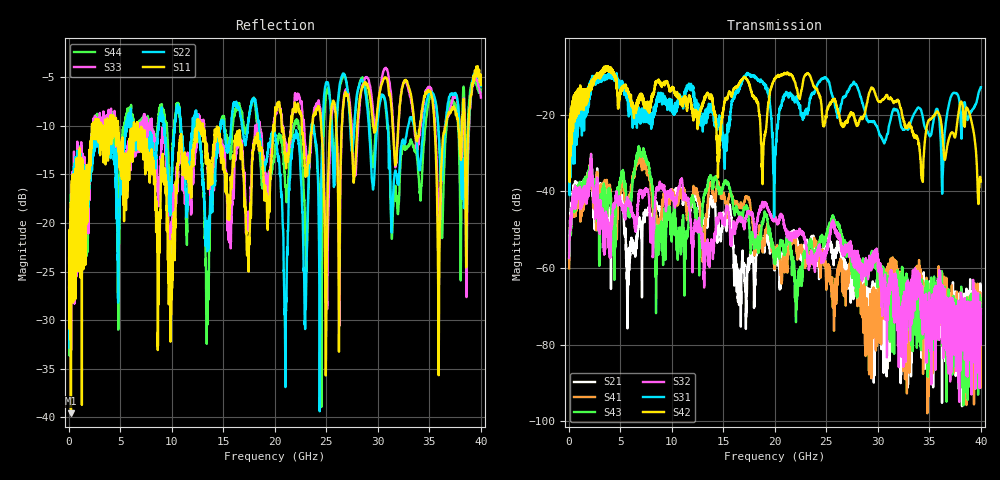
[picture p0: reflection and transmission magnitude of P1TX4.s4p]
!Agilent Technologies,N5245A,MY49151084,A.09.20.08
!Agilent N5245A: A.09.20.08
!Date: Thursday, March 01, 2012 14:23:38
!Correction: S11(Full 4 Port(1,2,3,4))
!S12(Full 4 Port(1,2,3,4))
!S13(Full 4 Port(1,2,3,4))
!S14(Full 4 Port(1,2,3,4))
!S21(Full 4 Port(1,2,3,4))
!S22(Full 4 Port(1,2,3,4))
!S23(Full 4 Port(1,2,3,4))
!S24(Full 4 Port(1,2,3,4))
!S31(Full 4 Port(1,2,3,4))
!S32(Full 4 Port(1,2,3,4))
!S33(Full 4 Port(1,2,3,4))
!S34(Full 4 Port(1,2,3,4))
!S41(Full 4 Port(1,2,3,4))
!S42(Full 4 Port(1,2,3,4))
!S43(Full 4 Port(1,2,3,4))
!S44(Full 4 Port(1,2,3,4))
!S4P File: Measurements: <S11,S12,S13,S14>,
!<S21,S22,S23,S24>,
!<S31,S32,S33,S34>,
!<S41,S42,S43,S44>:
# Hz S  dB  R 50
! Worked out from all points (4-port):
!   3996 points, 50 MHz to 40 GHz, reference 50 ohm
!   strongest paths, dB at 50 MHz, 10.04 GHz, 20.03 GHz, 30.02 GHz, 40 GHz:
!     S42: -25.4, -13.1, -10.5, -16.3, -37.4
!     S31: -26.4, -18.4, -30.0, -23.8, -12.8
!     S32: -57.3, -40.5, -47.3, -59.4, -70.7
!     S43: -56.1, -47.7, -59.1, -64.9, -71.9
!     S41: -60.1, -39.4, -56.6, -72.9, -69.0
!     S21: -57.8, -39.6, -59.7, -63.2, -66.5
!   lowest |S11| = -39.6 dB at 230 MHz (marker M1), VSWR 1.02, Z = 50.8 + j0.691 ohm
!   |S11| at or under -10 dB: start of sweep to 2.264 GHz; 6.674 GHz to 12.46 GHz (5.786 GHz wide, 60.5 % of centre); 13.03 GHz to 19.86 GHz (6.833 GHz wide, 41.6 % of centre)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
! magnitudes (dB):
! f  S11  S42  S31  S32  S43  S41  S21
! 50 MHz  -24.1  -25.4  -26.4  -57.3  -56.1  -60.1  -57.8
! 230 MHz  -39.6  -27.4  -31.2  -46.0  -46.6  -46.2  -44.3
! 6.92 GHz  -11.9  -14.6  -20.0  -39.6  -29.3  -31.3  -47.5
! 8.6 GHz  -23.0  -11.5  -15.6  -39.3  -49.2  -50.5  -44.0
! 13.72 GHz  -14.9  -15.6  -18.7  -54.9  -36.2  -37.8  -42.1
! 16.58 GHz  -10.7  -11.6  -13.3  -47.1  -45.7  -43.7  -65.3
! 40 GHz  -5.8  -37.4  -12.8  -70.7  -71.9  -69.0  -66.5
